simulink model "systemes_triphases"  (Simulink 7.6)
settings: Solver=ode23tb  StartTime=0.0  StopTime=0.2  RelTol=1e-3
undefined symbols (not defined in the file or in its folder): sigbuilder_block
libraries: powerlib x10, powerlib_extras x3

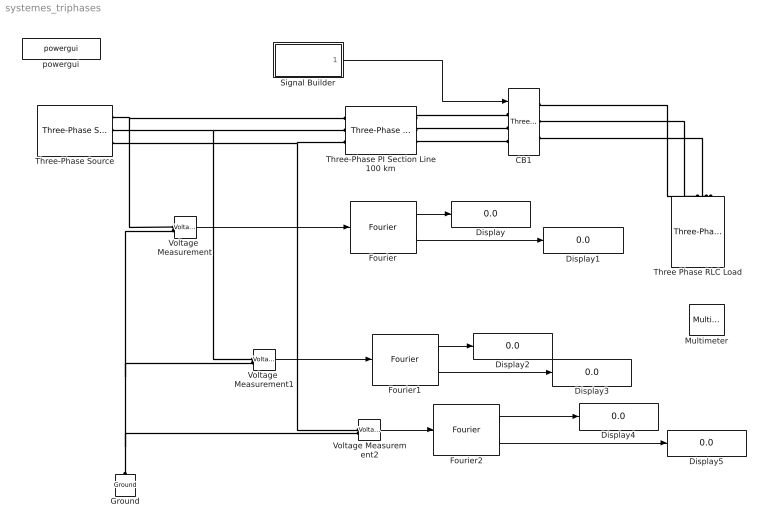
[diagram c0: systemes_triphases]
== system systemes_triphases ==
  CB1 : powerlib/Elements/Three-Phase Breaker  DialogController=POWERSYS.PowerSysDialog  SystemSampleTime=-1  InitialState=closed  SwitchA=on  SwitchB=on  SwitchC=on  SwitchTimes="[5/60  ]"  External=on  BreakerResistance=0.001  SnubberResistance=1e5  SnubberCapacitance=inf  Measurements=None
  Display{,1..5} (6 alike) : Display
  Fourier : powerlib_extras/Measurements/Fourier  DialogController=POWERSYS.PowerSysDialog  SystemSampleTime=-1  f1=60  n=1
  Fourier1 : powerlib_extras/Measurements/Fourier  DialogController=POWERSYS.PowerSysDialog  SystemSampleTime=-1  f1=60  n=1
  Fourier2 : powerlib_extras/Measurements/Fourier  DialogController=POWERSYS.PowerSysDialog  SystemSampleTime=-1  f1=60  n=1
  Ground : powerlib/Elements/Ground  DialogController=POWERSYS.PowerSysDialog  PhysicalDomain=powersysdomain  SubClassName=unknown  LeftPortType=p1  RightPortType=p1  LConnTagsString=a
  Multimeter : powerlib/Measurements/Multimeter  Tag=PoWeRsYsTeMmEaSuReMeNt  SystemSampleTime=-1  PhasorSimulation=off  OutputType=Magnitude  sel=[1 2 3]  L=3  Gain=[1 1 1]  yselected={'Uag: Three Phase RLC Load','Ubg: Three Phase RLC Load','Ucg: Three Phase RLC Load'};  PSBOutputType=1  PSBequivalent=0  AxesSetting=[0,0.1,-100,100]  Display=1  SavedBlockNames={}
  Signal Builder : Subsystem  Tag=STV Subsys  LoadFcn=sigbuilder_block('load');  StartFcn=sigbuilder_block('start');  StopFcn=sigbuilder_block('stop');  ClipboardFcn=sigbuilder_block('clipboard');
  Three Phase RLC Load : powerlib/Elements/Three-Phase Series RLC Load  DialogController=POWERSYS.PowerSysDialog  PhysicalDomain=powersysdomain  SubClassName=unknown  LeftPortType=p1  RightPortType=p1  LConnTagsString=A|B|C  Configuration=Y (grounded)  NominalVoltage=735e3  NominalFrequency=60  ActivePower=330e6/250  InductivePower=330e6  CapacitivePower=0  Measurements=Branch voltages
  Three-Phase PI Section Line 100 km : powerlib/Elements/Three-Phase PI Section Line  DialogController=POWERSYS.PowerSysDialog  PhysicalDomain=powersysdomain  SubClassName=unknown  LeftPortType=p1  RightPortType=p1  LConnTagsString=a|b|c  RConnTagsString=A|B|C  Frequency=60  Resistances=[ 0.01273 0.3864]  Inductances="[ 0.9337e-3  4.1264e-3]"  Capacitances=[12.74e-9 7.751e-9]  Length=100
  Three-Phase Source : powerlib/Electrical Sources/Three-Phase Source  DialogController=POWERSYS.PowerSysDialog  SystemSampleTime=-1  Voltage=25e3  PhaseAngle=0  Frequency=60  InternalConnection=Yg  SpecifyImpedance=on  Resistance=0.8929  Inductance=16.58e-3  ShortCircuitLevel=100e6  BaseVoltage=25e3  XRratio=7
  Voltage  Measurement : powerlib/Measurements/Voltage Measurement  DialogController=POWERSYS.PowerSysDialog  SystemSampleTime=-1  PhasorSimulation=off  OutputType=Complex  PSBequivalent=0
  Voltage  Measurement1 : powerlib/Measurements/Voltage Measurement  DialogController=POWERSYS.PowerSysDialog  SystemSampleTime=-1  PhasorSimulation=off  OutputType=Complex  PSBequivalent=0
  Voltage Measurement2 : powerlib/Measurements/Voltage Measurement  DialogController=POWERSYS.PowerSysDialog  SystemSampleTime=-1  PhasorSimulation=off  OutputType=Complex  PSBequivalent=0
  powergui : powerlib/powergui  SystemSampleTime=-1  SimulationMode=Continuous  SampleTime=0  frequency=60  SPID=off  DisableSnubberDevices=off  DisableRonSwitches=off  DisableVfSwitches=off  SwTol=0  Interpol=off  frequencyindice=0  echomessages=off  HookPort=off  DisplayEquations=off  FunctionMessages=off  EnableUseOfTLC=off  x0status=blocks  RestoreLinks=warning  ResistiveCurrentMeasurement=off  Frange=[0:2:500]  Ylog=off  Xlog=on  ShowGrid=off  save=off  variable=ZData  ZoomFFT=on  StartTime=0.0  cycles=1  DisplayStyle=1  fundamental=60  FreqAxis=off  MaxFrequency=1000  frequencyindicesteady=1  RmsSteady=1  display=off  Ts=0  methode=off
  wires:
  Signal Builder/1(Signal 2) -> CB1/1
  Voltage  Measurement/1 -> Fourier/1
  Fourier/1 -> Display/1
  Fourier/2 -> Display1/1
  Voltage  Measurement1/1 -> Fourier1/1
  Fourier1/1 -> Display2/1
  Fourier1/2 -> Display3/1
  Voltage Measurement2/1 -> Fourier2/1
  Fourier2/1 -> Display4/1
  Fourier2/2 -> Display5/1
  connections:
  Three-Phase Source/RConn1 -- Three-Phase PI Section Line 100 km/LConn1 -- Voltage  Measurement/LConn1
  Three-Phase Source/RConn2 -- Three-Phase PI Section Line 100 km/LConn2 -- Voltage  Measurement1/LConn1
  Three-Phase Source/RConn3 -- Three-Phase PI Section Line 100 km/LConn3 -- Voltage Measurement2/LConn1
  Three-Phase PI Section Line 100 km/RConn1 -- CB1/LConn1
  Three-Phase PI Section Line 100 km/RConn2 -- CB1/LConn2
  Three-Phase PI Section Line 100 km/RConn3 -- CB1/LConn3
  CB1/RConn1 -- Three Phase RLC Load/LConn1
  CB1/RConn2 -- Three Phase RLC Load/LConn2
  CB1/RConn3 -- Three Phase RLC Load/LConn3
  Ground/LConn1 -- Voltage  Measurement/LConn2 -- Voltage  Measurement1/LConn2 -- Voltage Measurement2/LConn2

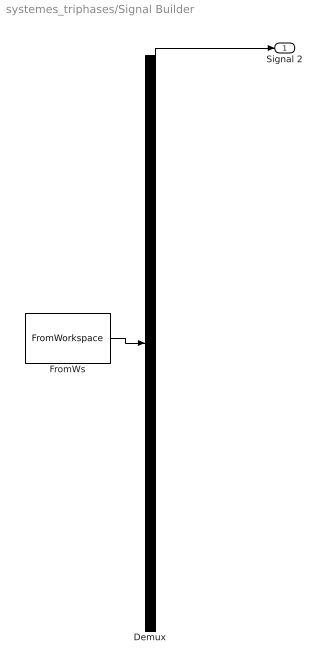
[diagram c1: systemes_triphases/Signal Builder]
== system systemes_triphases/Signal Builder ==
  Demux : Demux  Tag=STV Demux  Outputs=1
  FromWs : FromWorkspace  Tag=STV FromWs  VariableName=tuvar  SampleTime=0  SigBuilderData=DataTag0  VnvData=DataTag1
  Signal 2 : Outport  Tag=STV Outport
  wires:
  FromWs/1 -> Demux/1
  Demux/1 -> Signal 2/1
